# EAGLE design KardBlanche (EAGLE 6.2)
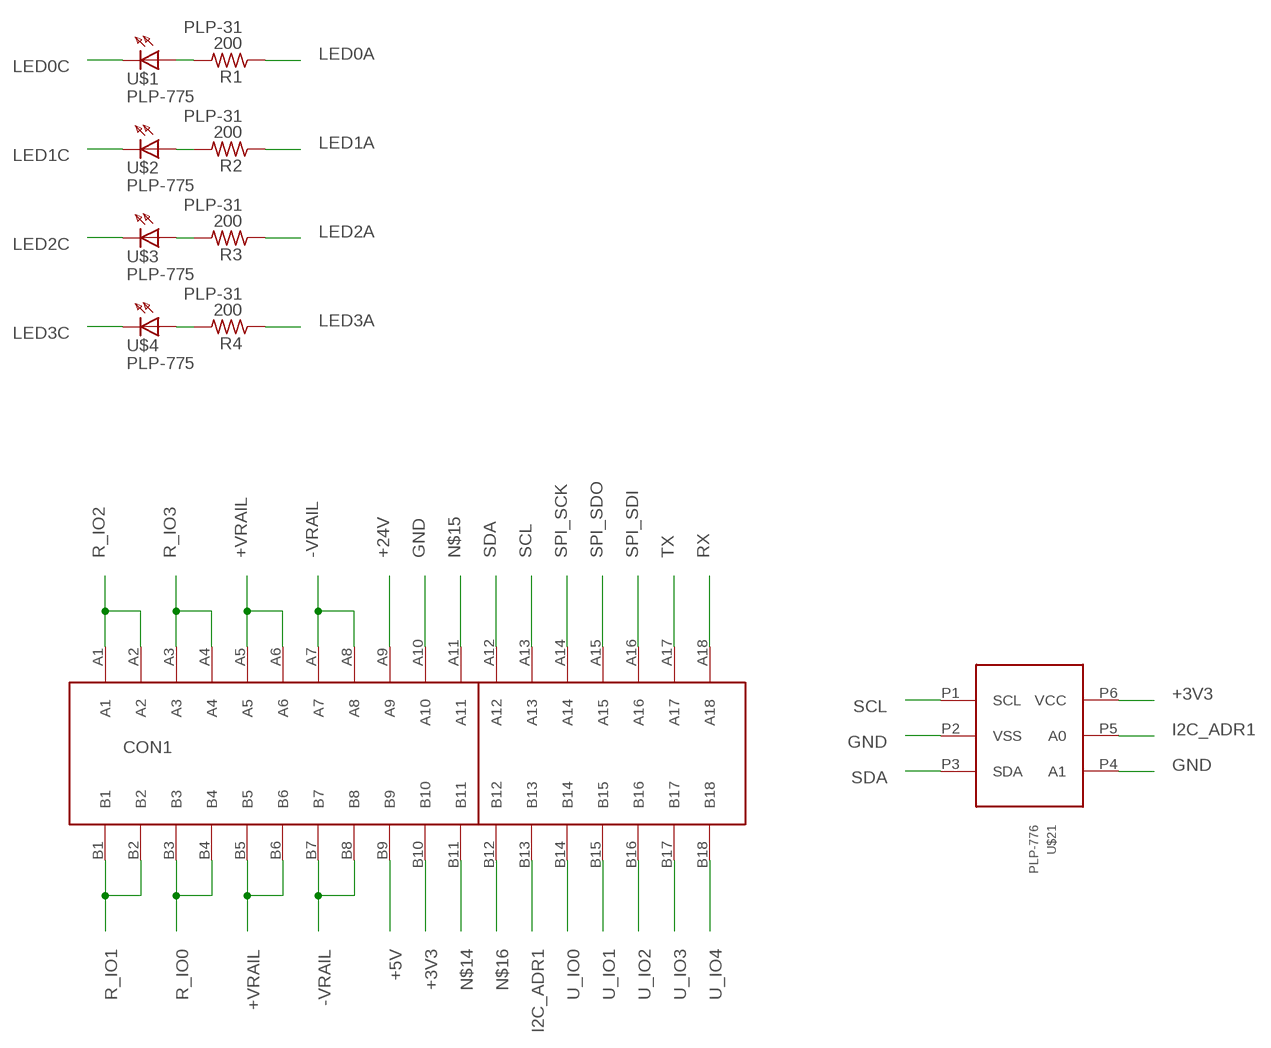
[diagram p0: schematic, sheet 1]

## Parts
CON1  PLPA-0105  [PLPA-0105]
R1  200  PLP-31  [DISCRETE_R0603]
R2  200  PLP-31  [DISCRETE_R0603]
R3  200  PLP-31  [DISCRETE_R0603]
R4  200  PLP-31  [DISCRETE_R0603]
U$1  PLP-775  [PLP-775]
U$2  PLP-775  [PLP-775]
U$3  PLP-775  [PLP-775]
U$4  PLP-775  [PLP-775]
U$21  PLP-776  [SOT23-6]

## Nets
+3V3: CON1.B10 U$21.P6(VCC)
+5V: CON1.B9
+24V: CON1.A9
+VRAIL: CON1.A5 CON1.A6 CON1.B5 CON1.B6
-VRAIL: CON1.A7 CON1.A8 CON1.B7 CON1.B8
GND: CON1.A10 U$21.P2(VSS) U$21.P4(A1)
I2C_ADR1: CON1.B13 U$21.P5(A0)
LED0A: R1.1
LED0C: U$1.C
LED1A: R2.1
LED1C: U$2.C
LED2A: R3.1
LED2C: U$3.C
LED3A: R4.1
LED3C: U$4.C
N$1: R1.2 U$1.A
N$2: R2.2 U$2.A
N$3: R3.2 U$3.A
N$4: R4.2 U$4.A
N$14: CON1.B11
N$15: CON1.A11
N$16: CON1.B12
R_IO0: CON1.B3 CON1.B4
R_IO1: CON1.B1 CON1.B2
R_IO2: CON1.A1 CON1.A2
R_IO3: CON1.A3 CON1.A4
RX: CON1.A18
SCL: CON1.A13 U$21.P1(SCL)
SDA: CON1.A12 U$21.P3(SDA)
SPI_SCK: CON1.A14
SPI_SDI: CON1.A16
SPI_SDO: CON1.A15
TX: CON1.A17
U_IO0: CON1.B14
U_IO1: CON1.B15
U_IO2: CON1.B16
U_IO3: CON1.B17
U_IO4: CON1.B18

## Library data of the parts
CON1 = PLP:PLPA-0105: CONN PCI EXPRESS 36POS VERT PCB; PLP#: PLPA-0105
R1-R4 = PLP:PLP-31: Resistor; PLP#: PLP-31
U$1-U$4 = PLP:PLP-775: LED Green RT Ang; PLP#: PLP-775
U$21 = PLP:PLP-776: IC EEPROM 2KBIT 400KHZ SOT23-6; PLP#: PLP-776

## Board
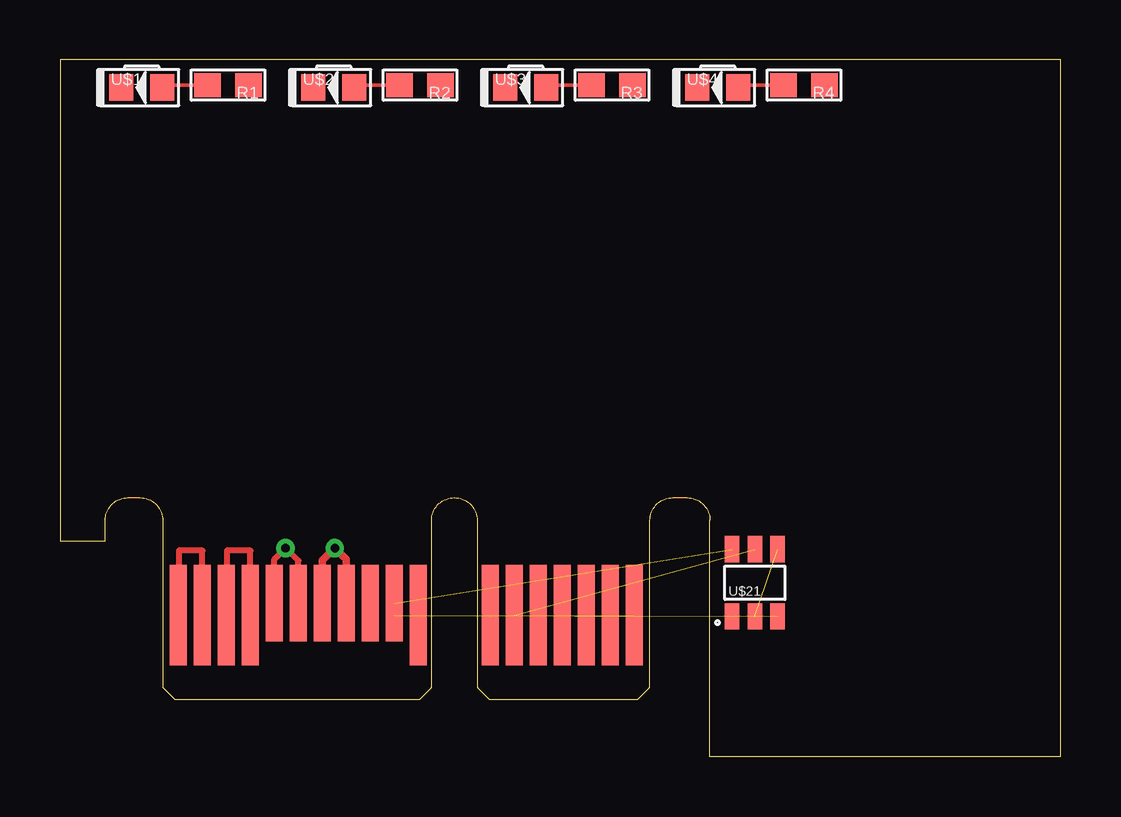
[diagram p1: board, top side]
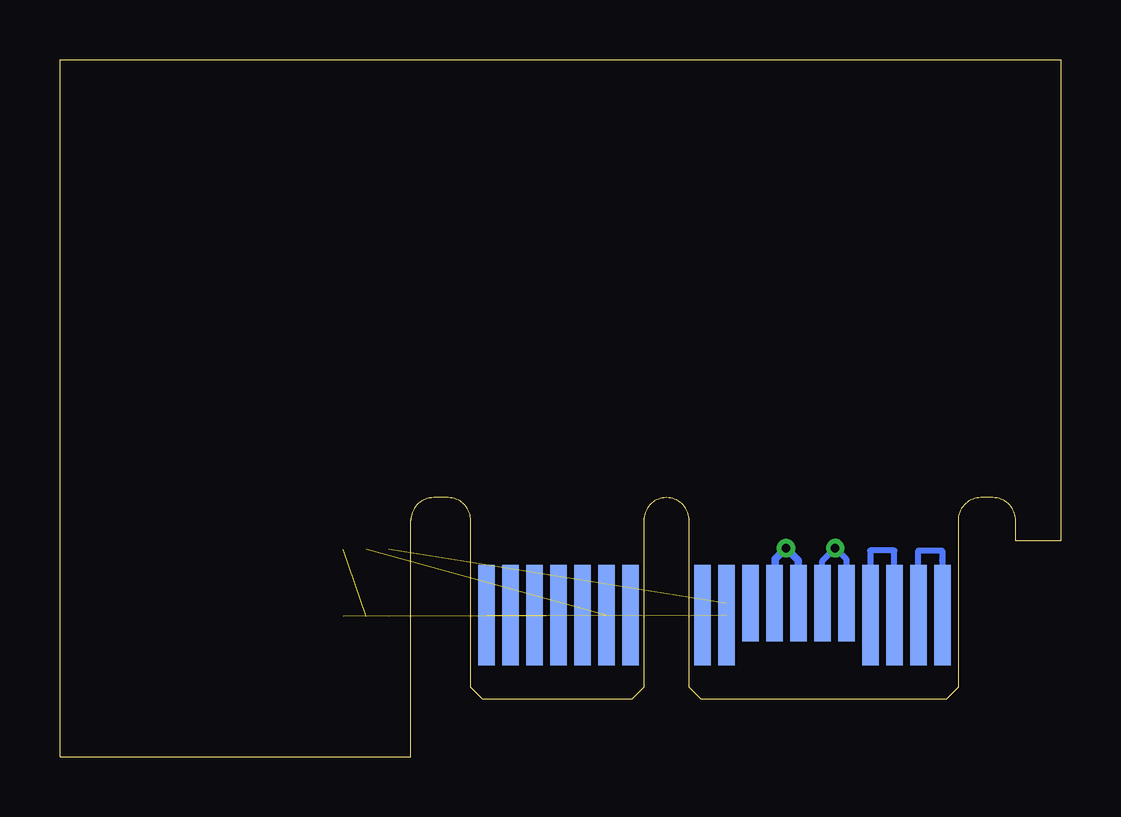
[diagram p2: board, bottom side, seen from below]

Size 41.7 x 29.05 mm. Coordinates in mm from the lower left corner, seen from the top.
Outline: 1.88,9.85 1.88,9 0,9 0,29.05 41.7,29.05 41.7,0 27.08,0 27.08,9.85
Copper layers (1*16): Top 0.0178mm / dielectric 59mil / Bottom 0.0178mm
Design rules: minimum track width 6mil, minimum drill 14mil, track to track 6mil, track to pad 6mil, pad to pad 6mil, via to via 6mil, smd to smd 6mil, copper to edge 20mil, drill to drill 16mil, minimum pad ring 8mil, minimum via ring 8mil, stop-mask expansion 3mil, vias tented up to drill 0mil, thermal gap 10mil
tKeepout: area 0,-1 to 0.8,29.1; area 41,-1 to 41.7,29.1
bKeepout: area 0,-1 to 0.8,29.1; area 41,-1 to 41.7,29.1

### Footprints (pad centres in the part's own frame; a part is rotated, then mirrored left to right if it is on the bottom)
PLPA-0105 = smd 0.7 x 4.2 bottom: A1 -11.5,3.5; A2 -10.5,3.5; A3 -9.5,3.5; A4 -8.5,3.5; A10 -2.5,3.5; A11 -1.5,3.5; A12 1.5,3.5; A13 2.5,3.5; A14 3.5,3.5; A15 4.5,3.5; A16 5.5,3.5; A17 6.5,3.5; A18 7.5,3.5 | smd 0.7 x 3.2 bottom: A5 -7.5,4; A6 -6.5,4; A7 -5.5,4; A8 -4.5,4; A9 -3.5,4 | smd 0.7 x 4.2: B1 -11.5,3.5; B2 -10.5,3.5; B3 -9.5,3.5; B4 -8.5,3.5; B11 -1.5,3.5; B12 1.5,3.5; B13 2.5,3.5; B14 3.5,3.5; B15 4.5,3.5; B16 5.5,3.5; B17 6.5,3.5; B18 7.5,3.5 | smd 0.7 x 3.2: B5 -7.5,4; B6 -6.5,4; B7 -5.5,4; B8 -4.5,4; B9 -3.5,4; B10 -2.5,4
DISCRETE_R0603 = smd 1.1 x 1: 1 -0.85,0; 2 0.85,0
PLP-775 = smd 1 x 1.1: A 0.85,0; C -0.85,0
SOT23-6 = smd 0.6 x 1.1: P1 -0.95,-1.4; P2 0,-1.4; P3 0.95,-1.4; P4 0.95,1.4; P5 0,1.4; P6 -0.95,1.4

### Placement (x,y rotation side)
CON1  16.43,2.4 0 top
R1  7,28 180 top
R2  15,28 180 top
R3  23,28 180 top
R4  31,28 180 top
U$1  3.4,27.9 0 top
U$2  11.4,27.9 0 top
U$3  19.4,27.9 0 top
U$4  27.4,27.9 0 top
U$21  28.95,7.25 0 top

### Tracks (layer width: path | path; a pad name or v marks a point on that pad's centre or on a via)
+3V3  (1 unrouted)
+VRAIL  (via drill 0.36)
  Top 0.254: CON1.A6 9.93,8.17 v9.4,8.7 8.93,8.23 CON1.A5
  Bottom 0.254: 8.95,7.85 8.95,8.25 v9.4,8.7 9.93,8.17 CON1.A6 | 8.95,7.85 8.95,7.8 | CON1.A5 8.95,5.92 8.95,7.85
-VRAIL  (via drill 0.36)
  Top 0.305: CON1.A7 10.93,8.18 v11.45,8.7 | CON1.A8 11.93,8.22 11.5,8.65 | 11.5,8.65 v11.45,8.7 | v11.45,8.7 11.5,8.65
  Bottom 0.305: CON1.A8 11.93,6.82 11.9,6.85 11.9,7 11.9,8.25 v11.45,8.7 10.93,8.18 CON1.A7
GND  (2 unrouted)
I2C_ADR1  (1 unrouted)
N$1
  Top 0.152: U$1.A 4.35,28 R1.2
N$2
  Top 0.152: U$2.A 12.35,28 R2.2
N$3
  Top 0.152: U$3.A 20.35,28 R3.2
N$4
  Top 0.152: U$4.A 28.35,28 R4.2
R_IO0
  Top 0.254: CON1.B4 7.93,8.6 6.95,8.6 CON1.B3
R_IO1
  Top 0.254: CON1.B2 5.93,8.6 4.95,8.6 CON1.B1
R_IO2
  Bottom 0.254: CON1.A2 5.93,8.6 4.95,8.6 4.95,8.2 CON1.A1
R_IO3
  Bottom 0.254: CON1.A3 6.93,8.6 7.95,8.6 CON1.A4
SCL  (1 unrouted)
SDA  (1 unrouted)

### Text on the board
Measures: TYP. | All dimensions are in mm. | Details of connector on page 4 of 10018784.pdf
